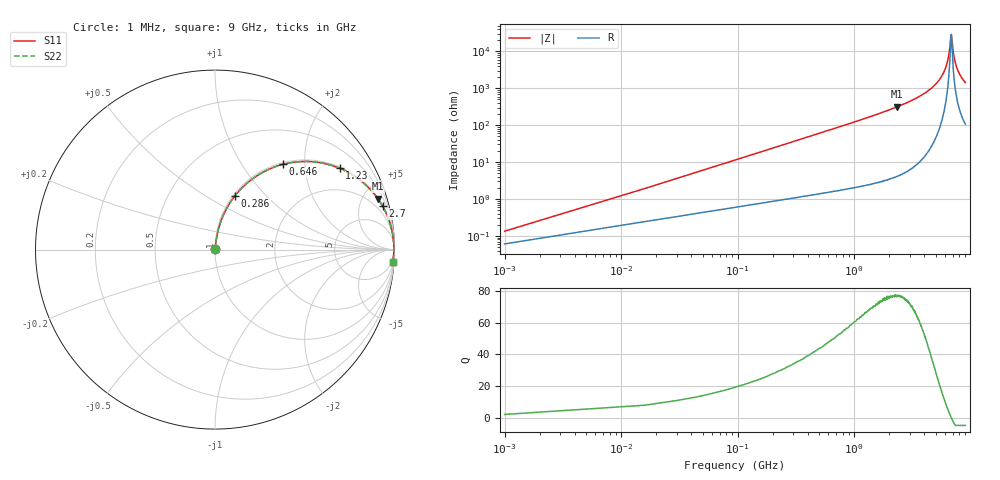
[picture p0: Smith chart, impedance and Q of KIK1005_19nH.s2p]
!version-3
!date-01.2023
!Series
# MHz S RI R 50
!Freq ReS11 ImS11 ReS21 ImS21 ReS12 ImS12 ReS22 ImS22
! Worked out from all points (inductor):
!   601 points, 1 MHz to 9 GHz, reference 50 ohm
!   read as one part in series: L = 19 nH near 46 MHz
!   highest Q = 77.2 at 2.34 GHz (marker M1), where L = 21.6 nH
!   self-resonance near 6.8 GHz
!   S11 on the Smith chart (normalised r, x): 1 MHz: 1.00, +0.00; 286 MHz: 1.02, +0.68; 646 MHz: 1.03, +1.56; 1.23 GHz: 1.05, +3.04; 2.7 GHz: 1.10, +7.66; 9 GHz: 3, -29
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1  0.00061 0.00119  0.9994 -0.00119  0.9994 -0.00119  0.00061 0.00119
61  0.00994 0.0718  0.9901 -0.0718  0.9901 -0.0718  0.00994 0.0718
76  0.0133 0.0891  0.9867 -0.0891  0.9867 -0.0891  0.0133 0.0891
151  0.0382 0.1722  0.9617 -0.1722  0.9617 -0.1722  0.0382 0.1722
286  0.112 0.3006  0.888 -0.3006  0.888 -0.3006  0.112 0.3006
646  0.3796 0.4753  0.6204 -0.4753  0.6204 -0.4753  0.3796 0.4753
1230  0.6951 0.4529  0.3049 -0.4529  0.3049 -0.4529  0.6951 0.4529
1520  0.7806 0.4068  0.2194 -0.4068  0.2194 -0.4068  0.7806 0.4068
2340  0.9065 0.2847  0.0935 -0.2847  0.0935 -0.2847  0.9065 0.2847
2700  0.9333 0.2429  0.0667 -0.2429  0.0667 -0.2429  0.9333 0.2429
3020  0.9499 0.2113  0.0501 -0.2113  0.0501 -0.2113  0.9499 0.2113
4520  0.9868 0.1021  0.0132 -0.1021  0.0132 -0.1021  0.9868 0.1021
5420  0.9941 0.0562  0.00595 -0.0562  0.00595 -0.0562  0.9941 0.0562
6020  0.9961 0.0302  0.00393 -0.0302  0.00393 -0.0302  0.9961 0.0302
6440  0.9966 0.0136  0.00342 -0.0136  0.00342 -0.0136  0.9966 0.0136
6800  0.9966 0.000292  0.00344 -0.000292  0.00344 -0.000292  0.9966 0.000292
6860  0.9965 -0.00186  0.00348 0.00186  0.00348 0.00186  0.9965 -0.00186
6990  0.9964 -0.00662  0.00361 0.00662  0.00361 0.00662  0.9964 -0.00662
7140  0.9962 -0.0118  0.00381 0.0118  0.00381 0.0118  0.9962 -0.0118
7520  0.9955 -0.0243  0.00453 0.0243  0.00453 0.0243  0.9955 -0.0243
8130  0.9937 -0.0436  0.00633 0.0436  0.00633 0.0436  0.9937 -0.0436
9000  0.99 -0.0687  0.00995 0.0687  0.00995 0.0687  0.99 -0.0687
